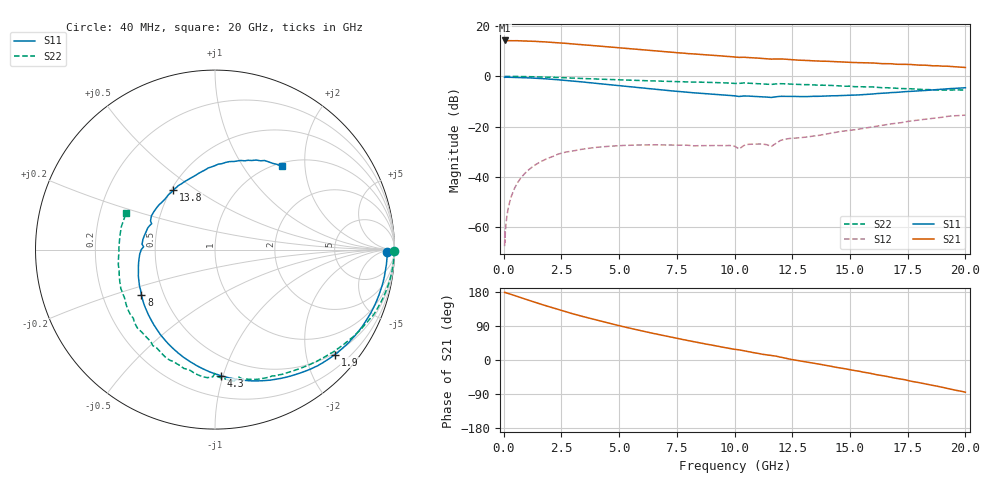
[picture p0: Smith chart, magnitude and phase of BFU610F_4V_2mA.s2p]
! Filename:  P:\Prog\Test\Noise\ATS_data\Testdata_Net\SplitFiles\BFU610_2W_A5_HighFreq_4V_2mA_D.s2p
! Date/Time: Wed 10/Aug/2011 16:57:43
! BFU610_2W_A5_HighFreq_4V_1mA_10mA_Bias2_R.s2p
! MDIF S-parameter v. bias file
! BFU610_2W_A5_HighFreq_4V_1mA_10mA
! Date/time Mon Aug 08 14:12:42 2011
! VAR V_out= 4.0010
! VAR I_out= 2.0000
! VAR V_in= 0.8618
! VAR I_in= 0.0145
! Device data file deembeded for feedlines and parallel
! Original file: \SplitFiles\BFU610_2W_A5_HighFreq_4V_2mA_R.s2p
! Feed-files: PR003V01_101208_Feed1.s2p, PR003V01_101208_Feed2.s2p
! Parallel-file: PR003V01_101208_Par.s2p
# MHz S MA R 50
!  Freq-MHz  S11-mag  S11-arg  S21-mag  S21-arg  S12-mag  S12-arg  S22-mag  S22-arg
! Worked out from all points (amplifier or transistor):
!   167 points, 40 MHz to 20 GHz, reference 50 ohm
!   highest |S21| = 14.3 dB at 40 MHz (marker M1)
!   |S21| within 3 dB of that: start of sweep to 5.076 GHz
!   unconditionally stable (mu >= 1): 6.975 GHz to 18.16 GHz
!   at 550 MHz: K = 0.00, MSG = 28.6 dB, |S12| = -43.1 dB
!   at 4.2 GHz: K = 0.49, MSG = 20.0 dB, |S12| = -28.0 dB
!   at 20 GHz: K = 0.85, MSG = 9.5 dB, |S12| = -15.4 dB
!   S11 on the Smith chart (normalised r, x): 40 MHz: 43, -15; 1.9 GHz: 0.47, -2.59; 4.3 GHz: 0.35, -0.99; 8 GHz: 0.37, -0.24; 13.8 GHz: 0.51, +0.41; 20 GHz: 1.06, +1.52
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40  0.9597 -0.8  5.163 178.4  0.0004234 85.1  0.9963 -0.3
50  0.9519 -1.3  5.137 178.7  0.0008647 52.4  0.997 -0.5
60  0.9596 -1.0  5.149 177.8  0.0005035 75.5  0.9973 -0.5
90  0.9597 -2.0  5.136 177.5  0.001062 88.5  0.9971 -0.9
200  0.9589 -4.5  5.104 175.6  0.002453 89.7  0.9971 -2.0
480  0.9539 -10.6  5.093 169.9  0.006104 86.4  0.9955 -5.0
1150  0.93 -25.3  5.01 156.4  0.01477 75.7  0.9846 -11.9
1900  0.8882 -41.2  4.795 141.7  0.02337 64.8  0.9648 -19.3
2700  0.8275 -57.4  4.523 127.1  0.03143 53.4  0.9333 -26.7
3400  0.7744 -70.7  4.251 115.3  0.03565 45.8  0.9081 -32.7
4300  0.7047 -87.1  3.932 101.0  0.03992 37.0  0.8762 -39.7
5400  0.6259 -106.1  3.554 84.8  0.04273 28.8  0.8416 -47.8
6800  0.5397 -129.2  3.133 66.1  0.04347 21.5  0.8032 -57.5
8000  0.4805 -148.6  2.828 51.1  0.04269 17.9  0.7727 -65.7
9400  0.4316 -170.4  2.553 34.8  0.04219 19.8  0.7464 -75.5
10200  0.3982 177.7  2.378 26.8  0.03606 22.2  0.7241 -79.3
12000  0.4009 152.2  2.215 7.4  0.05361 39.1  0.7149 -93.5
13400  0.4011 130.3  2.034 -8.3  0.06504 32.5  0.6748 -106.9
13800  0.4035 125.1  1.996 -12.4  0.06894 32.7  0.6651 -110.4
16800  0.4766 87.7  1.78 -45.9  0.114 19.4  0.5889 -145.8
18400  0.5304 69.7  1.649 -65.1  0.1432 6.1  0.5453 -171.0
20000  0.5944 51.4  1.5 -84.9  0.1701 -10.9  0.5345 157.6
